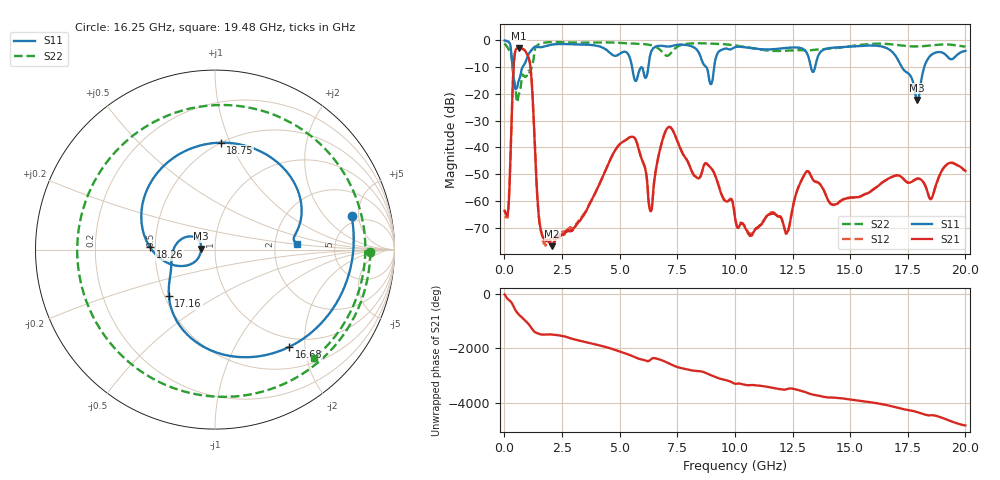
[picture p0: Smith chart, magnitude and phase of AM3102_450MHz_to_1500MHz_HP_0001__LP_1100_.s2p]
!Agilent Technologies,E8364B,MY43040894,A.07.50.67
!Agilent E8364B: A.07.50.67
!Date: Thursday, January 11, 2018 05:22:31
!Correction: S11(Full 2 Port(1,2))
!S21(Full 2 Port(1,2))
!S12(Full 2 Port(1,2))
!S22(Full 2 Port(1,2))
!S2P File: Measurements: S11, S21, S12, S22:
# Hz S  dB  R 50
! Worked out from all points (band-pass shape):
!   1601 points, 10 MHz to 20 GHz, reference 50 ohm
!   highest |S21| = -2.83 dB at 622.2 MHz (marker M1); lowest = -76.9 dB at 2.071 GHz (marker M2)
!   |S21| within 3 dB of the highest: 439.7 MHz to 1.017 GHz (577.3 MHz wide, 79.3 % of centre)
!   lowest |S11| = -22.3 dB at 17.91 GHz (marker M3), VSWR 1.17, Z = 42.9 + j0.429 ohm
!   |S11| at or under -10 dB: 354.9 MHz to 788.6 MHz (433.8 MHz wide, 75.9 % of centre); 5.539 GHz to 6.246 GHz (706.9 MHz wide, 12 % of centre); 17.24 GHz to 18.21 GHz (972.3 MHz wide, 5.48 % of centre)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
!   |S22| runs from -23.1 to -0.6 dB; largest |S21 - S12| = 0.003
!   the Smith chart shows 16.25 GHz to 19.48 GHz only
!   S11 on the Smith chart (normalised r, x): 16.25 GHz: 4.24, +4.06; 16.68 GHz: 0.84, -1.70; 17.16 GHz: 0.53, -0.31; 18.26 GHz: 0.47, +0.01; 18.75 GHz: 0.50, +0.92; 19.48 GHz: 2.67, +0.19
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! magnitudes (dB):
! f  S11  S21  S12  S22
! 10 MHz  -0.1  -63.7  -65.9  -1.1
! 434.8 MHz  -16.1  -6.2  -6.2  -15.8
! 622.2 MHz  -15.1  -2.8  -2.8  -20.4
! 1.109 GHz  -4.4  -8.7  -8.7  -12.0
! 1.597 GHz  -2.6  -71.6  -71.4  -1.2
! 2.071 GHz  -1.6  -76.9  -74.6  -0.7
! 3.346 GHz  -1.6  -66.6  -66.0  -0.9
! 5.07 GHz  -4.7  -38.3  -38.3  -1.0
! 6.332 GHz  -5.3  -63.8  -63.7  -1.7
! 6.682 GHz  -2.1  -43.4  -43.4  -3.0
! 7.219 GHz  -2.2  -32.6  -32.6  -4.8
! 10.01 GHz  -2.6  -66.1  -66.0  -1.9
! 12.25 GHz  -2.8  -72.1  -72.2  -3.9
! 13.34 GHz  -11.3  -51.4  -51.4  -3.6
! 16.25 GHz  -2.1  -54.1  -54.1  -1.3
! 16.68 GHz  -3.3  -51.6  -51.6  -1.4
! 17.16 GHz  -8.8  -50.7  -50.7  -1.9
! 17.91 GHz  -22.3  -51.6  -51.8  -2.3
! 18.26 GHz  -8.8  -54.3  -54.5  -2.1
! 18.75 GHz  -4.5  -53.3  -53.4  -1.7
! 19.48 GHz  -6.8  -46.0  -45.9  -1.7
! 20 GHz  -4.0  -48.8  -48.7  -2.4
